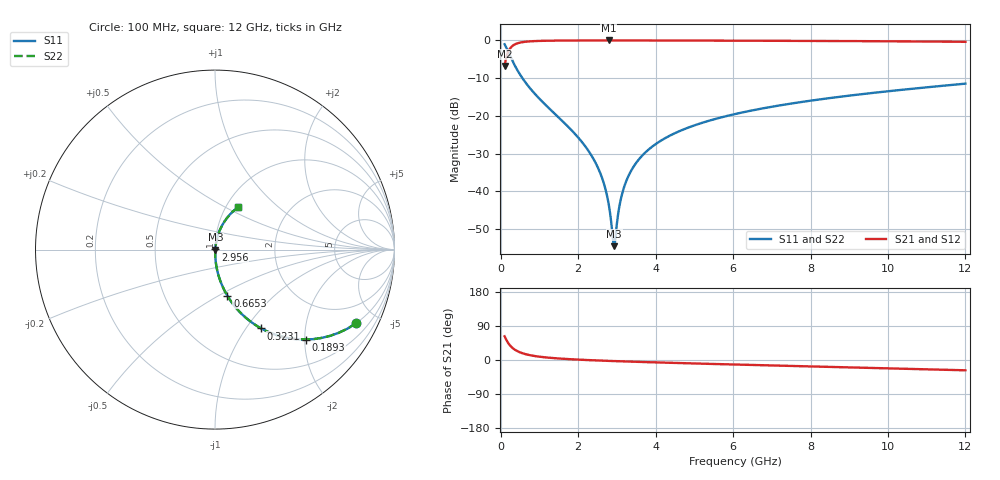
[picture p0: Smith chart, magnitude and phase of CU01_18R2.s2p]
! S-parameter model data by Modelithics Inc. support@modelithics.com 813-866-6335 Tampa FL USA
! S-Parameter data specifications:
! Substrate: 20-mil Rogers, substrate thickness, H=0.508mm, Dielectric constant, Er=3.75
! PCB Mounting Pad Footprint: Pad width, PadW=0.35mm , Pad length, PadL=0.30mm , Pad gap, PadG (edge-to-edge)=0.25mm , Reference planes=0.85mm apart
! Created Tue May  8 14:01:25 2018
# hz S ma R 50
! 2 Port Network Data from SP1.SP block
! freq  magS11  angS11  magS21  angS21  magS12  angS12  magS22  angS22
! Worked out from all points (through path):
!   801 points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, 100 MHz to 12 GHz, reference 50 ohm
!   highest |S21| = -0.02 dB at 2.792 GHz (marker M1); lowest = -6.8 dB at 100 MHz (marker M2)
!   group delay of S21, straight-line fit = 9.81 ps
!   lowest |S11| = -54.6 dB at 2.926 GHz (marker M3), VSWR 1.00, Z = 50.2 - j0.0176 ohm
!   |S11| at or under -10 dB: 559 MHz to end of sweep
!   |S22| runs from -54.6 to -1.0 dB; largest |S21 - S12| = 0
!   S11 on the Smith chart (normalised r, x): 100 MHz: 1.00, -3.85; 189.2 MHz: 1.00, -2.03; 323.1 MHz: 1.00, -1.18; 665.2 MHz: 1.00, -0.55; 2.956 GHz: 1.00, +0.00; 12 GHz: 1.14, +0.57
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1e8  0.888 -27.4  0.4594 62.5  0.4594 62.5  0.888 -27.4
1.8925e8  0.7132 -44.6  0.7003 45.3  0.7003 45.3  0.7132 -44.6
3.23125e8  0.5089 -59.6  0.8601 30.3  0.8601 30.3  0.5089 -59.6
4.57e8  0.3816 -67.9  0.9235 22.0  0.9235 22.0  0.3816 -67.9
6.6525e8  0.2658 -75.0  0.963 14.8  0.963 14.8  0.2658 -75.0
1.20075e9  0.1328 -83.0  0.9898 6.5  0.9898 6.5  0.1328 -83.0
2.09325e9  0.04521 -87.4  0.9973 0.5  0.9973 0.5  0.04521 -87.4
2.5395e9  0.01899 -86.1  0.998 -1.4  0.998 -1.4  0.01899 -86.1
2.68825e9  0.01147 -82.9  0.9981 -2.0  0.9981 -2.0  0.01147 -82.9
2.792375e9  0.006549 -76.1  0.9981 -2.4  0.9981 -2.4  0.006549 -76.1
2.881625e9  0.002817 -51.5  0.9981 -2.7  0.9981 -2.7  0.002817 -51.5
2.92625e9  0.00187 -5.4  0.9981 -2.9  0.9981 -2.9  0.00187 -5.4
2.956e9  0.002259 30.9  0.9981 -3.0  0.9981 -3.0  0.002259 30.9
3.10475e9  0.008003 72.7  0.998 -3.5  0.998 -3.5  0.008003 72.7
3.298125e9  0.01594 78.8  0.9979 -4.1  0.9979 -4.1  0.01594 78.8
3.6105e9  0.02808 80.7  0.9975 -5.1  0.9975 -5.1  0.02808 80.7
4.071625e9  0.04464 80.7  0.9968 -6.5  0.9968 -6.5  0.04464 80.7
4.88975e9  0.07128 79.3  0.995 -8.9  0.995 -8.9  0.07128 79.3
6.05e9  0.1055 76.6  0.9917 -12.0  0.9917 -12.0  0.1055 76.6
8.04325e9  0.1599 71.9  0.9839 -17.0  0.9839 -17.0  0.1599 71.9
1.002162e10  0.2123 67.0  0.9733 -22.0  0.9733 -22.0  0.2123 67.0
1.2e10  0.2671 61.6  0.9579 -27.2  0.9579 -27.2  0.2671 61.6
